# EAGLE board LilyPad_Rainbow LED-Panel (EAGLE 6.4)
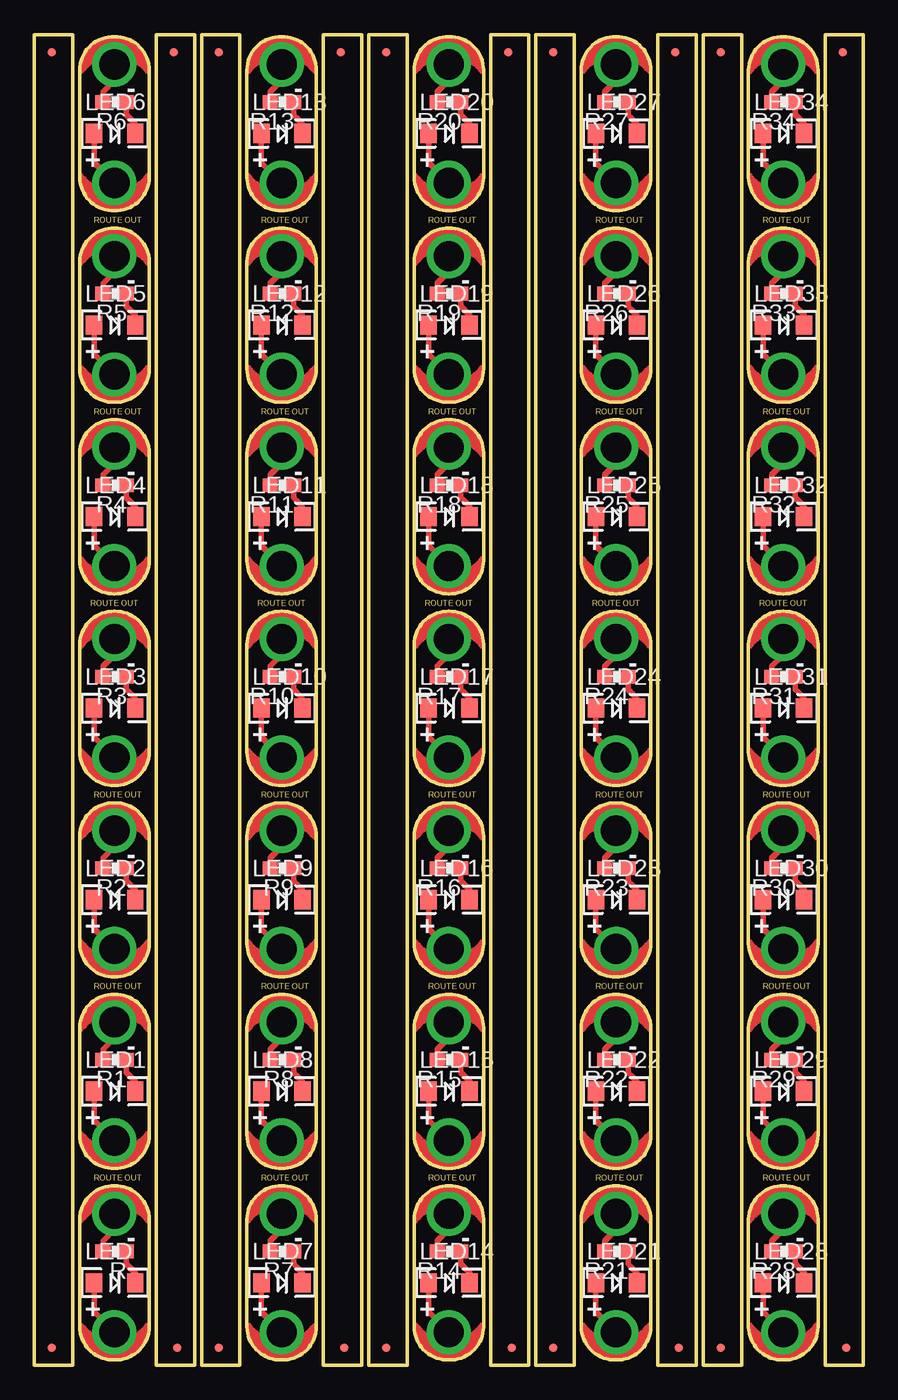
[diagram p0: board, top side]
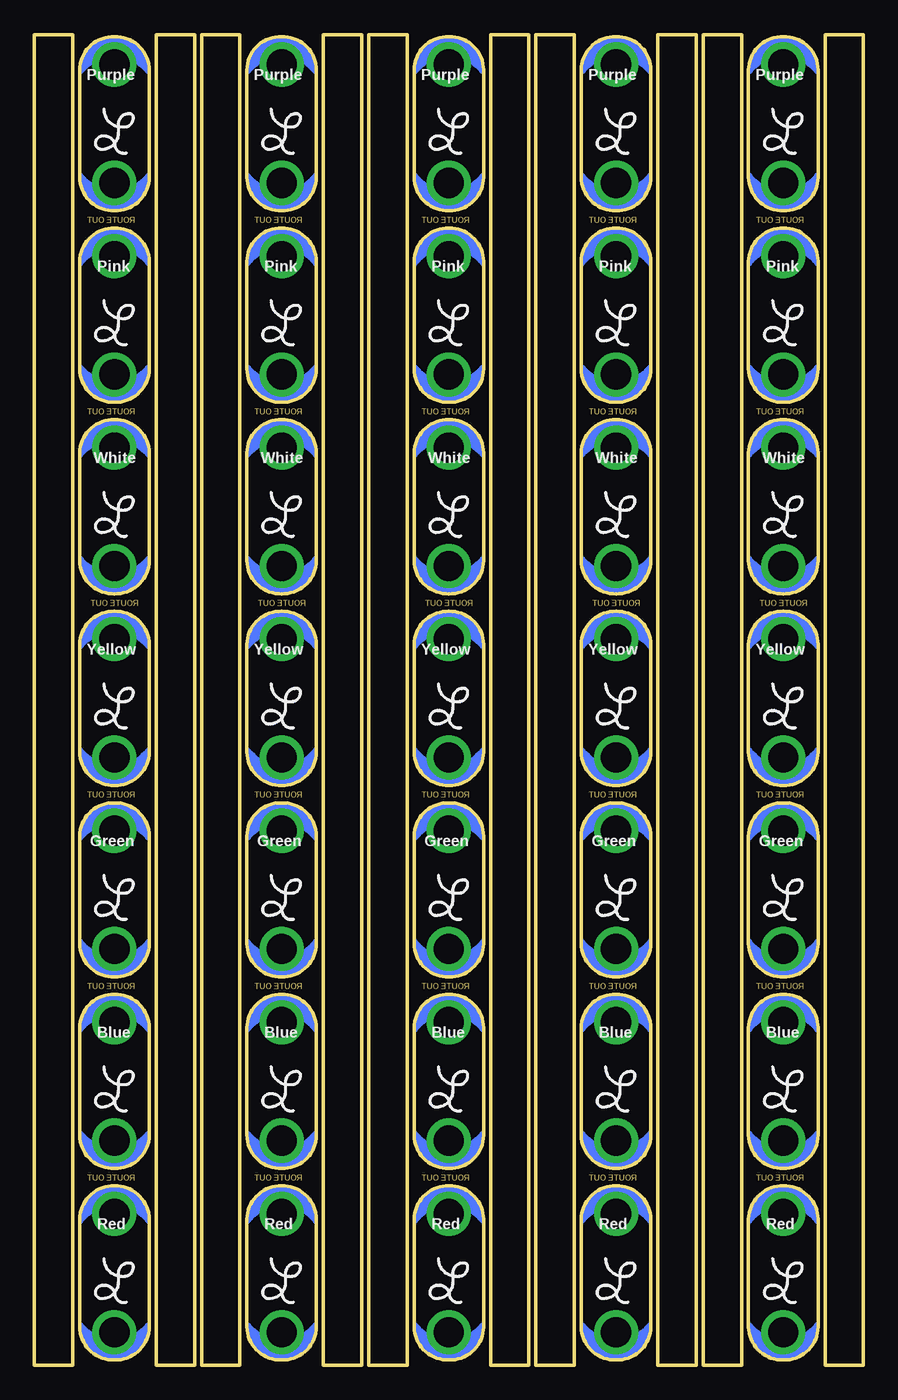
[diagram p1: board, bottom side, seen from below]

Size 60.45 x 97.03 mm. Coordinates in mm from the lower left corner, seen from the top.
Outline: 250 segments
Copper layers (1*16): Top 0.035mm / dielectric 1.5mm / Bottom 0.035mm
Design rules "SparkFun": minimum track width 8mil, minimum drill 20mil, track to track 8mil, track to pad 8mil, pad to pad 8mil, via to via 8mil, smd to smd 8mil, copper to edge 8mil, drill to drill 8mil, minimum pad ring 12mil, minimum via ring 10mil, stop-mask expansion 4mil, vias tented up to drill 20mil, thermal gap 10mil

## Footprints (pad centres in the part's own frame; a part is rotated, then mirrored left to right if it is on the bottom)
MICRO-FIDUCIAL = smd 0.635 x 0.635: 1 0,0
LED-1206 = smd 1.2 x 1.4: A -1.5,0; C 1.5,0
PETAL-SMALL = drill 2.2: 1 0,0
0603-RES = smd 1.1 x 1: 1 -0.85,0; 2 0.85,0

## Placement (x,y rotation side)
E$1  [MICRO-FIDUCIAL]  1.27,95.76 0 top
E$2  [MICRO-FIDUCIAL]  10.16,95.76 0 top
E$3  [MICRO-FIDUCIAL]  1.27,1.27 0 top
E$4  [MICRO-FIDUCIAL]  10.41,1.27 0 top
E$5  [MICRO-FIDUCIAL]  13.46,95.76 0 top
E$6  [MICRO-FIDUCIAL]  22.35,95.76 0 top
E$7  [MICRO-FIDUCIAL]  13.46,1.27 0 top
E$8  [MICRO-FIDUCIAL]  22.61,1.27 0 top
E$9  [MICRO-FIDUCIAL]  25.65,95.76 0 top
E$10  [MICRO-FIDUCIAL]  34.54,95.76 0 top
E$11  [MICRO-FIDUCIAL]  25.65,1.27 0 top
E$12  [MICRO-FIDUCIAL]  34.8,1.27 0 top
E$13  [MICRO-FIDUCIAL]  37.85,95.76 0 top
E$14  [MICRO-FIDUCIAL]  46.74,95.76 0 top
E$15  [MICRO-FIDUCIAL]  37.85,1.27 0 top
E$16  [MICRO-FIDUCIAL]  46.99,1.27 0 top
E$17  [MICRO-FIDUCIAL]  50.04,95.76 0 top
E$18  [MICRO-FIDUCIAL]  58.93,95.76 0 top
E$19  [MICRO-FIDUCIAL]  50.04,1.27 0 top
E$20  [MICRO-FIDUCIAL]  59.18,1.27 0 top
LED  White  [LED-1206]  5.86,6.02 0 top
LED1  White  [LED-1206]  5.86,19.99 0 top
LED2  White  [LED-1206]  5.86,33.96 0 top
LED3  White  [LED-1206]  5.86,47.93 0 top
LED4  White  [LED-1206]  5.86,61.9 0 top
LED5  White  [LED-1206]  5.86,75.87 0 top
LED6  White  [LED-1206]  5.86,89.84 0 top
LED7  White  [LED-1206]  18.05,6.02 0 top
LED8  White  [LED-1206]  18.05,19.99 0 top
LED9  White  [LED-1206]  18.05,33.96 0 top
LED10  White  [LED-1206]  18.05,47.93 0 top
LED11  White  [LED-1206]  18.05,61.9 0 top
LED12  White  [LED-1206]  18.05,75.87 0 top
LED13  White  [LED-1206]  18.05,89.84 0 top
LED14  White  [LED-1206]  30.25,6.02 0 top
LED15  White  [LED-1206]  30.25,19.99 0 top
LED16  White  [LED-1206]  30.25,33.96 0 top
LED17  White  [LED-1206]  30.25,47.93 0 top
LED18  White  [LED-1206]  30.25,61.9 0 top
LED19  White  [LED-1206]  30.25,75.87 0 top
LED20  White  [LED-1206]  30.25,89.84 0 top
LED21  White  [LED-1206]  42.44,6.02 0 top
LED22  White  [LED-1206]  42.44,19.99 0 top
LED23  White  [LED-1206]  42.44,33.96 0 top
LED24  White  [LED-1206]  42.44,47.93 0 top
LED25  White  [LED-1206]  42.44,61.9 0 top
LED26  White  [LED-1206]  42.44,75.87 0 top
LED27  White  [LED-1206]  42.44,89.84 0 top
LED28  White  [LED-1206]  54.63,6.02 0 top
LED29  White  [LED-1206]  54.63,19.99 0 top
LED30  White  [LED-1206]  54.63,33.96 0 top
LED31  White  [LED-1206]  54.63,47.93 0 top
LED32  White  [LED-1206]  54.63,61.9 0 top
LED33  White  [LED-1206]  54.63,75.87 0 top
LED34  White  [LED-1206]  54.63,89.84 0 top
LED+  SEWTAP6  [PETAL-SMALL]  5.84,2.41 0 top
LED+1  SEWTAP6  [PETAL-SMALL]  5.84,16.38 0 top
LED+2  SEWTAP6  [PETAL-SMALL]  5.84,30.35 0 top
LED+3  SEWTAP6  [PETAL-SMALL]  5.84,44.32 0 top
LED+4  SEWTAP6  [PETAL-SMALL]  5.84,58.29 0 top
LED+5  SEWTAP6  [PETAL-SMALL]  5.84,72.26 0 top
LED+6  SEWTAP6  [PETAL-SMALL]  5.84,86.23 0 top
LED+7  SEWTAP6  [PETAL-SMALL]  18.03,2.41 0 top
LED+8  SEWTAP6  [PETAL-SMALL]  18.03,16.38 0 top
LED+9  SEWTAP6  [PETAL-SMALL]  18.03,30.35 0 top
LED+10  SEWTAP6  [PETAL-SMALL]  18.03,44.32 0 top
LED+11  SEWTAP6  [PETAL-SMALL]  18.03,58.29 0 top
LED+12  SEWTAP6  [PETAL-SMALL]  18.03,72.26 0 top
LED+13  SEWTAP6  [PETAL-SMALL]  18.03,86.23 0 top
LED+14  SEWTAP6  [PETAL-SMALL]  30.23,2.41 0 top
LED+15  SEWTAP6  [PETAL-SMALL]  30.23,16.38 0 top
LED+16  SEWTAP6  [PETAL-SMALL]  30.23,30.35 0 top
LED+17  SEWTAP6  [PETAL-SMALL]  30.23,44.32 0 top
LED+18  SEWTAP6  [PETAL-SMALL]  30.23,58.29 0 top
LED+19  SEWTAP6  [PETAL-SMALL]  30.23,72.26 0 top
LED+20  SEWTAP6  [PETAL-SMALL]  30.23,86.23 0 top
LED+21  SEWTAP6  [PETAL-SMALL]  42.42,2.41 0 top
LED+22  SEWTAP6  [PETAL-SMALL]  42.42,16.38 0 top
LED+23  SEWTAP6  [PETAL-SMALL]  42.42,30.35 0 top
LED+24  SEWTAP6  [PETAL-SMALL]  42.42,44.32 0 top
LED+25  SEWTAP6  [PETAL-SMALL]  42.42,58.29 0 top
LED+26  SEWTAP6  [PETAL-SMALL]  42.42,72.26 0 top
LED+27  SEWTAP6  [PETAL-SMALL]  42.42,86.23 0 top
LED+28  SEWTAP6  [PETAL-SMALL]  54.61,2.41 0 top
LED+29  SEWTAP6  [PETAL-SMALL]  54.61,16.38 0 top
LED+30  SEWTAP6  [PETAL-SMALL]  54.61,30.35 0 top
LED+31  SEWTAP6  [PETAL-SMALL]  54.61,44.32 0 top
LED+32  SEWTAP6  [PETAL-SMALL]  54.61,58.29 0 top
LED+33  SEWTAP6  [PETAL-SMALL]  54.61,72.26 0 top
LED+34  SEWTAP6  [PETAL-SMALL]  54.61,86.23 0 top
LED-  SEWTAP6  [PETAL-SMALL]  5.84,11.05 180 top
LED-1  SEWTAP6  [PETAL-SMALL]  5.84,25.02 180 top
LED-2  SEWTAP6  [PETAL-SMALL]  5.84,38.99 180 top
LED-3  SEWTAP6  [PETAL-SMALL]  5.84,52.96 180 top
LED-4  SEWTAP6  [PETAL-SMALL]  5.84,66.93 180 top
LED-5  SEWTAP6  [PETAL-SMALL]  5.84,80.9 180 top
LED-6  SEWTAP6  [PETAL-SMALL]  5.84,94.87 180 top
LED-7  SEWTAP6  [PETAL-SMALL]  18.03,11.05 180 top
LED-8  SEWTAP6  [PETAL-SMALL]  18.03,25.02 180 top
LED-9  SEWTAP6  [PETAL-SMALL]  18.03,38.99 180 top
LED-10  SEWTAP6  [PETAL-SMALL]  18.03,52.96 180 top
LED-11  SEWTAP6  [PETAL-SMALL]  18.03,66.93 180 top
LED-12  SEWTAP6  [PETAL-SMALL]  18.03,80.9 180 top
LED-13  SEWTAP6  [PETAL-SMALL]  18.03,94.87 180 top
LED-14  SEWTAP6  [PETAL-SMALL]  30.23,11.05 180 top
LED-15  SEWTAP6  [PETAL-SMALL]  30.23,25.02 180 top
LED-16  SEWTAP6  [PETAL-SMALL]  30.23,38.99 180 top
LED-17  SEWTAP6  [PETAL-SMALL]  30.23,52.96 180 top
LED-18  SEWTAP6  [PETAL-SMALL]  30.23,66.93 180 top
LED-19  SEWTAP6  [PETAL-SMALL]  30.23,80.9 180 top
LED-20  SEWTAP6  [PETAL-SMALL]  30.23,94.87 180 top
LED-21  SEWTAP6  [PETAL-SMALL]  42.42,11.05 180 top
LED-22  SEWTAP6  [PETAL-SMALL]  42.42,25.02 180 top
LED-23  SEWTAP6  [PETAL-SMALL]  42.42,38.99 180 top
LED-24  SEWTAP6  [PETAL-SMALL]  42.42,52.96 180 top
LED-25  SEWTAP6  [PETAL-SMALL]  42.42,66.93 180 top
LED-26  SEWTAP6  [PETAL-SMALL]  42.42,80.9 180 top
LED-27  SEWTAP6  [PETAL-SMALL]  42.42,94.87 180 top
LED-28  SEWTAP6  [PETAL-SMALL]  54.61,11.05 180 top
LED-29  SEWTAP6  [PETAL-SMALL]  54.61,25.02 180 top
LED-30  SEWTAP6  [PETAL-SMALL]  54.61,38.99 180 top
LED-31  SEWTAP6  [PETAL-SMALL]  54.61,52.96 180 top
LED-32  SEWTAP6  [PETAL-SMALL]  54.61,66.93 180 top
LED-33  SEWTAP6  [PETAL-SMALL]  54.61,80.9 180 top
LED-34  SEWTAP6  [PETAL-SMALL]  54.61,94.87 180 top
LOGO1  LOGO-LPL  [LOGO-L]  5.84,6.17 0 bottom
LOGO2  LOGO-LPL  [LOGO-L]  5.84,20.14 0 bottom
LOGO3  LOGO-LPL  [LOGO-L]  5.84,34.11 0 bottom
LOGO4  LOGO-LPL  [LOGO-L]  5.84,48.08 0 bottom
LOGO5  LOGO-LPL  [LOGO-L]  5.84,62.05 0 bottom
LOGO6  LOGO-LPL  [LOGO-L]  5.84,76.02 0 bottom
LOGO7  LOGO-LPL  [LOGO-L]  5.84,89.99 0 bottom
LOGO8  LOGO-LPL  [LOGO-L]  18.03,6.17 0 bottom
LOGO9  LOGO-LPL  [LOGO-L]  18.03,20.14 0 bottom
LOGO10  LOGO-LPL  [LOGO-L]  18.03,34.11 0 bottom
LOGO11  LOGO-LPL  [LOGO-L]  18.03,48.08 0 bottom
LOGO12  LOGO-LPL  [LOGO-L]  18.03,62.05 0 bottom
LOGO13  LOGO-LPL  [LOGO-L]  18.03,76.02 0 bottom
LOGO14  LOGO-LPL  [LOGO-L]  18.03,89.99 0 bottom
LOGO15  LOGO-LPL  [LOGO-L]  30.23,6.17 0 bottom
LOGO16  LOGO-LPL  [LOGO-L]  30.23,20.14 0 bottom
LOGO17  LOGO-LPL  [LOGO-L]  30.23,34.11 0 bottom
LOGO18  LOGO-LPL  [LOGO-L]  30.23,48.08 0 bottom
LOGO19  LOGO-LPL  [LOGO-L]  30.23,62.05 0 bottom
LOGO20  LOGO-LPL  [LOGO-L]  30.23,76.02 0 bottom
LOGO21  LOGO-LPL  [LOGO-L]  30.23,89.99 0 bottom
LOGO22  LOGO-LPL  [LOGO-L]  42.42,6.17 0 bottom
LOGO23  LOGO-LPL  [LOGO-L]  42.42,20.14 0 bottom
LOGO24  LOGO-LPL  [LOGO-L]  42.42,34.11 0 bottom
LOGO25  LOGO-LPL  [LOGO-L]  42.42,48.08 0 bottom
LOGO26  LOGO-LPL  [LOGO-L]  42.42,62.05 0 bottom
LOGO27  LOGO-LPL  [LOGO-L]  42.42,76.02 0 bottom
LOGO28  LOGO-LPL  [LOGO-L]  42.42,89.99 0 bottom
LOGO29  LOGO-LPL  [LOGO-L]  54.61,6.17 0 bottom
LOGO30  LOGO-LPL  [LOGO-L]  54.61,20.14 0 bottom
LOGO31  LOGO-LPL  [LOGO-L]  54.61,34.11 0 bottom
LOGO32  LOGO-LPL  [LOGO-L]  54.61,48.08 0 bottom
LOGO33  LOGO-LPL  [LOGO-L]  54.61,62.05 0 bottom
LOGO34  LOGO-LPL  [LOGO-L]  54.61,76.02 0 bottom
LOGO35  LOGO-LPL  [LOGO-L]  54.61,89.99 0 bottom
R  100  [0603-RES]  5.86,8.3 180 top
R1  100  [0603-RES]  5.86,22.27 180 top
R2  100  [0603-RES]  5.86,36.25 180 top
R3  100  [0603-RES]  5.86,50.22 180 top
R4  100  [0603-RES]  5.86,64.19 180 top
R5  100  [0603-RES]  5.86,78.16 180 top
R6  100  [0603-RES]  5.86,92.12 180 top
R7  100  [0603-RES]  18.05,8.3 180 top
R8  100  [0603-RES]  18.05,22.27 180 top
R9  100  [0603-RES]  18.05,36.25 180 top
R10  100  [0603-RES]  18.05,50.22 180 top
R11  100  [0603-RES]  18.05,64.19 180 top
R12  100  [0603-RES]  18.05,78.16 180 top
R13  100  [0603-RES]  18.05,92.12 180 top
R14  100  [0603-RES]  30.25,8.3 180 top
R15  100  [0603-RES]  30.25,22.27 180 top
R16  100  [0603-RES]  30.25,36.25 180 top
R17  100  [0603-RES]  30.25,50.22 180 top
R18  100  [0603-RES]  30.25,64.19 180 top
R19  100  [0603-RES]  30.25,78.16 180 top
R20  100  [0603-RES]  30.25,92.12 180 top
R21  100  [0603-RES]  42.44,8.3 180 top
R22  100  [0603-RES]  42.44,22.27 180 top
R23  100  [0603-RES]  42.44,36.25 180 top
R24  100  [0603-RES]  42.44,50.22 180 top
R25  100  [0603-RES]  42.44,64.19 180 top
R26  100  [0603-RES]  42.44,78.16 180 top
R27  100  [0603-RES]  42.44,92.12 180 top
R28  100  [0603-RES]  54.63,8.3 180 top
R29  100  [0603-RES]  54.63,22.27 180 top
R30  100  [0603-RES]  54.63,36.25 180 top
R31  100  [0603-RES]  54.63,50.22 180 top
R32  100  [0603-RES]  54.63,64.19 180 top
R33  100  [0603-RES]  54.63,78.16 180 top
R34  100  [0603-RES]  54.63,92.12 180 top

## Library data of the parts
E$1-E$20 = SparkFun-Aesthetics
LED LED1-LED34 = SparkFun-3-2-07
LED+ LED+1-LED+34 LED- LED-1-LED-34 LOGO1-LOGO35 = LilyPad-Wearables
R R1-R34 = SparkFun

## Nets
+: LED+.1 LED.A
+1: LED1.A LED+1.1
+2: LED2.A LED+2.1
+3: LED3.A LED+3.1
+4: LED4.A LED+4.1
+5: LED5.A LED+5.1
+6: LED6.A LED+6.1
+7: LED7.A LED+7.1
+8: LED8.A LED+8.1
+9: LED9.A LED+9.1
+10: LED10.A LED+10.1
+11: LED11.A LED+11.1
+12: LED12.A LED+12.1
+13: LED13.A LED+13.1
+14: LED14.A LED+14.1
+15: LED15.A LED+15.1
+16: LED16.A LED+16.1
+17: LED17.A LED+17.1
+18: LED18.A LED+18.1
+19: LED19.A LED+19.1
+20: LED20.A LED+20.1
+21: LED21.A LED+21.1
+22: LED22.A LED+22.1
+23: LED23.A LED+23.1
+24: LED24.A LED+24.1
+25: LED25.A LED+25.1
+26: LED26.A LED+26.1
+27: LED27.A LED+27.1
+28: LED28.A LED+28.1
+29: LED29.A LED+29.1
+30: LED30.A LED+30.1
+31: LED31.A LED+31.1
+32: LED32.A LED+32.1
+33: LED33.A LED+33.1
+34: LED34.A LED+34.1
-: LED-.1 R.2
-1: LED-1.1 R1.2
-2: LED-2.1 R2.2
-3: LED-3.1 R3.2
-4: LED-4.1 R4.2
-5: LED-5.1 R5.2
-6: LED-6.1 R6.2
-7: LED-7.1 R7.2
-8: LED-8.1 R8.2
-9: LED-9.1 R9.2
-10: LED-10.1 R10.2
-11: LED-11.1 R11.2
-12: LED-12.1 R12.2
-13: LED-13.1 R13.2
-14: LED-14.1 R14.2
-15: LED-15.1 R15.2
-16: LED-16.1 R16.2
-17: LED-17.1 R17.2
-18: LED-18.1 R18.2
-19: LED-19.1 R19.2
-20: LED-20.1 R20.2
-21: LED-21.1 R21.2
-22: LED-22.1 R22.2
-23: LED-23.1 R23.2
-24: LED-24.1 R24.2
-25: LED-25.1 R25.2
-26: LED-26.1 R26.2
-27: LED-27.1 R27.2
-28: LED-28.1 R28.2
-29: LED-29.1 R29.2
-30: LED-30.1 R30.2
-31: LED-31.1 R31.2
-32: LED-32.1 R32.2
-33: LED-33.1 R33.2
-34: LED-34.1 R34.2
N$1: LED.C R.1
N$2: LED1.C R1.1
N$3: LED2.C R2.1
N$4: LED3.C R3.1
N$5: LED4.C R4.1
N$6: LED5.C R5.1
N$7: LED6.C R6.1
N$8: LED7.C R7.1
N$9: LED8.C R8.1
N$10: LED9.C R9.1
N$11: LED10.C R10.1
N$12: LED11.C R11.1
N$13: LED12.C R12.1
N$14: LED13.C R13.1
N$15: LED14.C R14.1
N$16: LED15.C R15.1
N$17: LED16.C R16.1
N$18: LED17.C R17.1
N$19: LED18.C R18.1
N$20: LED19.C R19.1
N$21: LED20.C R20.1
N$22: LED21.C R21.1
N$23: LED22.C R22.1
N$24: LED23.C R23.1
N$25: LED24.C R24.1
N$26: LED25.C R25.1
N$27: LED26.C R26.1
N$28: LED27.C R27.1
N$29: LED28.C R28.1
N$30: LED29.C R29.1
N$31: LED30.C R30.1
N$32: LED31.C R31.1
N$33: LED32.C R32.1
N$34: LED33.C R33.1
N$35: LED34.C R34.1

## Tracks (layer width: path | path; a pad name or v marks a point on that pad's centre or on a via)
+
  Top 0.406: 5.84,2.29 LED+.1 4.36,3.89 LED.A
+1
  Top 0.406: 5.84,16.26 LED+1.1 4.36,17.86 LED1.A
+2
  Top 0.406: 5.84,30.23 LED+2.1 4.36,31.83 LED2.A
+3
  Top 0.406: 5.84,44.2 LED+3.1 4.36,45.8 LED3.A
+4
  Top 0.406: 5.84,58.17 LED+4.1 4.36,59.77 LED4.A
+5
  Top 0.406: 5.84,72.14 LED+5.1 4.36,73.74 LED5.A
+6
  Top 0.406: 5.84,86.11 LED+6.1 4.36,87.71 LED6.A
+7
  Top 0.406: 18.03,2.29 LED+7.1 16.55,3.89 LED7.A
+8
  Top 0.406: 18.03,16.26 LED+8.1 16.55,17.86 LED8.A
+9
  Top 0.406: 18.03,30.23 LED+9.1 16.55,31.83 LED9.A
+10
  Top 0.406: 18.03,44.2 LED+10.1 16.55,45.8 LED10.A
+11
  Top 0.406: 18.03,58.17 LED+11.1 16.55,59.77 LED11.A
+12
  Top 0.406: 18.03,72.14 LED+12.1 16.55,73.74 LED12.A
+13
  Top 0.406: 18.03,86.11 LED+13.1 16.55,87.71 LED13.A
+14
  Top 0.406: 30.23,2.29 LED+14.1 28.75,3.89 LED14.A
+15
  Top 0.406: 30.23,16.26 LED+15.1 28.75,17.86 LED15.A
+16
  Top 0.406: 30.23,30.23 LED+16.1 28.75,31.83 LED16.A
+17
  Top 0.406: 30.23,44.2 LED+17.1 28.75,45.8 LED17.A
+18
  Top 0.406: 30.23,58.17 LED+18.1 28.75,59.77 LED18.A
+19
  Top 0.406: 30.23,72.14 LED+19.1 28.75,73.74 LED19.A
+20
  Top 0.406: 30.23,86.11 LED+20.1 28.75,87.71 LED20.A
+21
  Top 0.406: 42.42,2.29 LED+21.1 40.94,3.89 LED21.A
+22
  Top 0.406: 42.42,16.26 LED+22.1 40.94,17.86 LED22.A
+23
  Top 0.406: 42.42,30.23 LED+23.1 40.94,31.83 LED23.A
+24
  Top 0.406: 42.42,44.2 LED+24.1 40.94,45.8 LED24.A
+25
  Top 0.406: 42.42,58.17 LED+25.1 40.94,59.77 LED25.A
+26
  Top 0.406: 42.42,72.14 LED+26.1 40.94,73.74 LED26.A
+27
  Top 0.406: 42.42,86.11 LED+27.1 40.94,87.71 LED27.A
+28
  Top 0.406: 54.61,2.29 LED+28.1 53.13,3.89 LED28.A
+29
  Top 0.406: 54.61,16.26 LED+29.1 53.13,17.86 LED29.A
+30
  Top 0.406: 54.61,30.23 LED+30.1 53.13,31.83 LED30.A
+31
  Top 0.406: 54.61,44.2 LED+31.1 53.13,45.8 LED31.A
+32
  Top 0.406: 54.61,58.17 LED+32.1 53.13,59.77 LED32.A
+33
  Top 0.406: 54.61,72.14 LED+33.1 53.13,73.74 LED33.A
+34
  Top 0.406: 54.61,86.11 LED+34.1 53.13,87.71 LED34.A
-
  Top 0.406: LED-.1 5.84,9.91 5.01,9.08 R.2
-1
  Top 0.406: LED-1.1 5.84,23.88 5.01,23.05 R1.2
-2
  Top 0.406: LED-2.1 5.84,37.85 5.01,37.02 R2.2
-3
  Top 0.406: LED-3.1 5.84,51.82 5.01,50.99 R3.2
-4
  Top 0.406: LED-4.1 5.84,65.79 5.01,64.96 R4.2
-5
  Top 0.406: LED-5.1 5.84,79.76 5.01,78.93 R5.2
-6
  Top 0.406: LED-6.1 5.84,93.73 5.01,92.9 R6.2
-7
  Top 0.406: LED-7.1 18.03,9.91 17.2,9.08 R7.2
-8
  Top 0.406: LED-8.1 18.03,23.88 17.2,23.05 R8.2
-9
  Top 0.406: LED-9.1 18.03,37.85 17.2,37.02 R9.2
-10
  Top 0.406: LED-10.1 18.03,51.82 17.2,50.99 R10.2
-11
  Top 0.406: LED-11.1 18.03,65.79 17.2,64.96 R11.2
-12
  Top 0.406: LED-12.1 18.03,79.76 17.2,78.93 R12.2
-13
  Top 0.406: LED-13.1 18.03,93.73 17.2,92.9 R13.2
-14
  Top 0.406: LED-14.1 30.23,9.91 29.4,9.08 R14.2
-15
  Top 0.406: LED-15.1 30.23,23.88 29.4,23.05 R15.2
-16
  Top 0.406: LED-16.1 30.23,37.85 29.4,37.02 R16.2
-17
  Top 0.406: LED-17.1 30.23,51.82 29.4,50.99 R17.2
-18
  Top 0.406: LED-18.1 30.23,65.79 29.4,64.96 R18.2
-19
  Top 0.406: LED-19.1 30.23,79.76 29.4,78.93 R19.2
-20
  Top 0.406: LED-20.1 30.23,93.73 29.4,92.9 R20.2
-21
  Top 0.406: LED-21.1 42.42,9.91 41.59,9.08 R21.2
-22
  Top 0.406: LED-22.1 42.42,23.88 41.59,23.05 R22.2
-23
  Top 0.406: LED-23.1 42.42,37.85 41.59,37.02 R23.2
-24
  Top 0.406: LED-24.1 42.42,51.82 41.59,50.99 R24.2
-25
  Top 0.406: LED-25.1 42.42,65.79 41.59,64.96 R25.2
-26
  Top 0.406: LED-26.1 42.42,79.76 41.59,78.93 R26.2
-27
  Top 0.406: LED-27.1 42.42,93.73 41.59,92.9 R27.2
-28
  Top 0.406: LED-28.1 54.61,9.91 53.78,9.08 R28.2
-29
  Top 0.406: LED-29.1 54.61,23.88 53.78,23.05 R29.2
-30
  Top 0.406: LED-30.1 54.61,37.85 53.78,37.02 R30.2
-31
  Top 0.406: LED-31.1 54.61,51.82 53.78,50.99 R31.2
-32
  Top 0.406: LED-32.1 54.61,65.79 53.78,64.96 R32.2
-33
  Top 0.406: LED-33.1 54.61,79.76 53.78,78.93 R33.2
-34
  Top 0.406: LED-34.1 54.61,93.73 53.78,92.9 R34.2
N$1
  Top 0.254: 6.92,7.17 6.86,7.24
  Top 0.406: LED.C 7.36,6.74 6.92,7.17 6.71,7.38 R.1
N$2
  Top 0.254: 6.92,21.15 6.86,21.21
  Top 0.406: LED1.C 7.36,20.7 6.92,21.15 6.71,21.36 R1.1
N$3
  Top 0.254: 6.92,35.12 6.86,35.18
  Top 0.406: LED2.C 7.36,34.67 6.92,35.12 6.71,35.33 R2.1
N$4
  Top 0.254: 6.92,49.08 6.86,49.15
  Top 0.406: LED3.C 7.36,48.64 6.92,49.08 6.71,49.3 R3.1
N$5
  Top 0.254: 6.92,63.06 6.86,63.12
  Top 0.406: LED4.C 7.36,62.61 6.92,63.06 6.71,63.27 R4.1
N$6
  Top 0.254: 6.92,77.03 6.86,77.09
  Top 0.406: LED5.C 7.36,76.59 6.92,77.03 6.71,77.23 R5.1
N$7
  Top 0.254: 6.92,91 6.86,91.06
  Top 0.406: LED6.C 7.36,90.56 6.92,91 6.71,91.2 R6.1
N$8
  Top 0.254: 19.11,7.17 19.05,7.24
  Top 0.406: LED7.C 19.55,6.74 19.11,7.17 18.9,7.38 R7.1
N$9
  Top 0.254: 19.11,21.15 19.05,21.21
  Top 0.406: LED8.C 19.55,20.7 19.11,21.15 18.9,21.36 R8.1
N$10
  Top 0.254: 19.11,35.12 19.05,35.18
  Top 0.406: LED9.C 19.55,34.67 19.11,35.12 18.9,35.33 R9.1
N$11
  Top 0.254: 19.11,49.08 19.05,49.15
  Top 0.406: LED10.C 19.55,48.64 19.11,49.08 18.9,49.3 R10.1
N$12
  Top 0.254: 19.11,63.06 19.05,63.12
  Top 0.406: LED11.C 19.55,62.61 19.11,63.06 18.9,63.27 R11.1
N$13
  Top 0.254: 19.11,77.03 19.05,77.09
  Top 0.406: LED12.C 19.55,76.59 19.11,77.03 18.9,77.23 R12.1
N$14
  Top 0.254: 19.11,91 19.05,91.06
  Top 0.406: LED13.C 19.55,90.56 19.11,91 18.9,91.2 R13.1
N$15
  Top 0.254: 31.3,7.17 31.24,7.24
  Top 0.406: LED14.C 31.75,6.74 31.3,7.17 31.1,7.38 R14.1
N$16
  Top 0.254: 31.3,21.15 31.24,21.21
  Top 0.406: LED15.C 31.75,20.7 31.3,21.15 31.1,21.36 R15.1
N$17
  Top 0.254: 31.3,35.12 31.24,35.18
  Top 0.406: LED16.C 31.75,34.67 31.3,35.12 31.1,35.33 R16.1
N$18
  Top 0.254: 31.3,49.08 31.24,49.15
  Top 0.406: LED17.C 31.75,48.64 31.3,49.08 31.1,49.3 R17.1
N$19
  Top 0.254: 31.3,63.06 31.24,63.12
  Top 0.406: LED18.C 31.75,62.61 31.3,63.06 31.1,63.27 R18.1
N$20
  Top 0.254: 31.3,77.03 31.24,77.09
  Top 0.406: LED19.C 31.75,76.59 31.3,77.03 31.1,77.23 R19.1
N$21
  Top 0.254: 31.3,91 31.24,91.06
  Top 0.406: LED20.C 31.75,90.56 31.3,91 31.1,91.2 R20.1
N$22
  Top 0.254: 43.5,7.17 43.43,7.24
  Top 0.406: LED21.C 43.94,6.74 43.5,7.17 43.29,7.38 R21.1
N$23
  Top 0.254: 43.5,21.15 43.43,21.21
  Top 0.406: LED22.C 43.94,20.7 43.5,21.15 43.29,21.36 R22.1
N$24
  Top 0.254: 43.5,35.12 43.43,35.18
  Top 0.406: LED23.C 43.94,34.67 43.5,35.12 43.29,35.33 R23.1
N$25
  Top 0.254: 43.5,49.08 43.43,49.15
  Top 0.406: LED24.C 43.94,48.64 43.5,49.08 43.29,49.3 R24.1
N$26
  Top 0.254: 43.5,63.06 43.43,63.12
  Top 0.406: LED25.C 43.94,62.61 43.5,63.06 43.29,63.27 R25.1
N$27
  Top 0.254: 43.5,77.03 43.43,77.09
  Top 0.406: LED26.C 43.94,76.59 43.5,77.03 43.29,77.23 R26.1
N$28
  Top 0.254: 43.5,91 43.43,91.06
  Top 0.406: LED27.C 43.94,90.56 43.5,91 43.29,91.2 R27.1
N$29
  Top 0.254: 55.69,7.17 55.63,7.24
  Top 0.406: LED28.C 56.13,6.74 55.69,7.17 55.48,7.38 R28.1
N$30
  Top 0.254: 55.69,21.15 55.63,21.21
  Top 0.406: LED29.C 56.13,20.7 55.69,21.15 55.48,21.36 R29.1
N$31
  Top 0.254: 55.69,35.12 55.63,35.18
  Top 0.406: LED30.C 56.13,34.67 55.69,35.12 55.48,35.33 R30.1
N$32
  Top 0.254: 55.69,49.08 55.63,49.15
  Top 0.406: LED31.C 56.13,48.64 55.69,49.08 55.48,49.3 R31.1
N$33
  Top 0.254: 55.69,63.06 55.63,63.12
  Top 0.406: LED32.C 56.13,62.61 55.69,63.06 55.48,63.27 R32.1
N$34
  Top 0.254: 55.69,77.03 55.63,77.09
  Top 0.406: LED33.C 56.13,76.59 55.69,77.03 55.48,77.23 R33.1
N$35
  Top 0.254: 55.69,91 55.63,91.06
  Top 0.406: LED34.C 56.13,90.56 55.69,91 55.48,91.2 R34.1

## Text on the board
Dimension: One vertical strip equal 1 unit. This is a panel of 5 'boards' | ROUTE OUT | ROUTE OUT | ROUTE OUT | ROUTE OUT | ROUTE OUT | ROUTE OUT | ROUTE OUT | ROUTE OUT | ROUTE OUT | ROUTE OUT | ROUTE OUT | ROUTE OUT | ROUTE OUT | ROUTE OUT | ROUTE OUT | ROUTE OUT | ROUTE OUT | ROUTE OUT | ROUTE OUT | ROUTE OUT | ROUTE OUT | ROUTE OUT | ROUTE OUT | ROUTE OUT | ROUTE OUT | ROUTE OUT | ROUTE OUT | ROUTE OUT | ROUTE OUT | ROUTE OUT
tPlace: - | - | - | - | - | + | + | + | + | + | - | - | - | - | - | + | + | + | + | + | - | - | - | - | - | + | + | + | + | + | - | - | - | - | - | + | + | + | + | + | - | - | - | - | - | + | + | + | + | + | - | - | - | - | - | + | + | + | + | + | - | - | - | - | - | + | + | + | + | +
bPlace: Purple | Purple | Purple | Purple | Purple | Pink | Pink | Pink | Pink | Pink | White | White | White | White | White | Yellow | Yellow | Yellow | Yellow | Yellow | Green | Green | Green | Green | Green | Blue | Blue | Blue | Blue | Blue | Red | Red | Red | Red | Red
